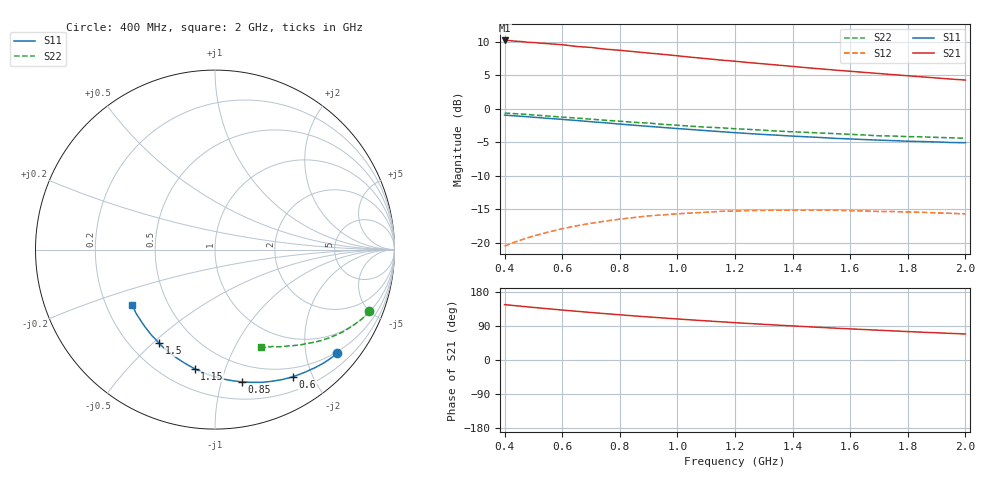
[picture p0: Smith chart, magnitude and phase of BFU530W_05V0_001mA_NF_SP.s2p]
! Filename:  P:\Prog\Test\Noise\ATS_data\Testdata_Net\06 Compressed Noise after Statistics\BFU530W_APM2013_09_A05_05p0V_001mA_NF_CM01_D.sf
! Date/Time: Tue 26/Mar/2013 18:06:06
! BFU530W_APM2013_09_A05_05p0V_1to25mA_NF_CM01_Bias1_R.sf
! Noise Parameter Data File
! BFU530W_APM2013_09_A05_05p0V_1to25mA_NF_CM01
! Date/time: Thu Mar 21 20:31:54 2013
! freq range =  0.4000 to  2.0000 GHz, 37 points
! bias range =  0.9950 to 25.0000 mA, 9 points
! bias supplies used: 1 1 0 0 0 0
! VAR bias_mode= 1  ! Specify V_out, I_out
! VAR bias_var = 1  ! Bias variable = I_out
! VAR V_out= 5.000000
! VAR I_out= 0.995000
! VAR V_in= 0.782600
! VAR I_in= 0.010101
! Device data file deembeded for feedlines and parallel
! Original file: \06 Compressed Noise after Statistics\BFU530W_APM2013_09_A05_05p0V_001mA_NF_CM01_R.sf
! Feed-files: PR019V01_070313_Feed1.s2p, PR019V01_070313_Feed2.s2p
! Parallel-file: PR019V01_070313_Par.s2p
# MHz S MA R 50
!  Freq-MHz  S11-mag  S11-arg  S21-mag  S21-arg  S12-mag  S12-arg  S22-mag  S22-arg
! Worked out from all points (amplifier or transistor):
!   37 points, 400 MHz to 2 GHz, reference 50 ohm
!   highest |S21| = 10.2 dB at 400 MHz (marker M1)
!   |S21| within 3 dB of that: start of sweep to 1.172 GHz
!   unconditionally stable (mu >= 1): nowhere
!   at 500 MHz: K = 0.20, MSG = 14.4 dB, |S12| = -19.0 dB
!   at 1.1 GHz: K = 0.41, MSG = 11.5 dB, |S12| = -15.5 dB
!   at 2 GHz: K = 0.77, MSG = 10.0 dB, |S12| = -15.7 dB
!   lowest NFmin = 0.48 dB at 420 MHz
!   S11 on the Smith chart (normalised r, x): 400 MHz: 0.46, -2.66; 600 MHz: 0.38, -1.72; 850 MHz: 0.34, -1.16; 1.15 GHz: 0.33, -0.79; 1.5 GHz: 0.32, -0.52; 2 GHz: 0.31, -0.28
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400  0.8945 -40.3  3.224 146.2  0.09419 64.3  0.9268 -21.8
420  0.8877 -42.2  3.212 144.6  0.09802 63.2  0.9211 -22.7
460  0.876 -46.0  3.163 141.7  0.1053 61.0  0.9099 -24.6
480  0.8694 -47.7  3.124 140.2  0.1087 59.9  0.9036 -25.5
500  0.8625 -49.6  3.111 138.7  0.112 58.9  0.8964 -26.3
600  0.8311 -58.5  2.998 131.8  0.127 54.0  0.8642 -30.5
650  0.8154 -62.6  2.908 128.6  0.1337 51.8  0.8504 -32.3
700  0.7982 -66.9  2.858 125.3  0.1395 49.5  0.834 -34.3
750  0.7834 -70.8  2.776 122.3  0.1449 47.6  0.8189 -35.9
800  0.7668 -74.7  2.723 119.3  0.1498 45.7  0.805 -37.6
850  0.7514 -78.7  2.659 116.4  0.1541 43.8  0.7903 -39.2
950  0.7236 -86.0  2.541 110.9  0.1611 40.4  0.7636 -42.2
1050  0.6977 -93.0  2.415 105.7  0.1665 37.4  0.7388 -44.9
1150  0.6732 -99.7  2.303 100.9  0.1713 34.7  0.7197 -47.2
1200  0.6618 -102.9  2.256 98.5  0.1721 33.5  0.7078 -48.7
1250  0.6512 -106.0  2.202 96.3  0.1739 32.3  0.6995 -49.6
1350  0.633 -112.1  2.11 92.0  0.1745 30.4  0.6796 -52.1
1500  0.6082 -120.8  1.977 85.9  0.1749 27.7  0.6574 -55.3
1600  0.5941 -126.4  1.899 82.1  0.1733 26.4  0.6429 -57.4
1750  0.577 -134.1  1.792 76.8  0.1707 25.2  0.6242 -60.2
1850  0.568 -139.1  1.724 73.4  0.1685 24.5  0.6158 -62.1
2000  0.557 -146.4  1.633 68.6  0.1638 24.5  0.6015 -65.0
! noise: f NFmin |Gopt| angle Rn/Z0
400  0.5358  0.6261  24.36  0.3103
460  0.5234  0.6349  27.94  0.3332
600  0.5889  0.6383  37.14  0.3289
800  0.543  0.6261  49.28  0.2894
1000  0.6921  0.6502  61.41  0.3076
1200  0.7441  0.6335  74.71  0.255
1400  0.788  0.6208  89.12  0.2023
1600  0.7562  0.5474  99.32  0.1568
1800  0.8933  0.5797  114.5  0.1448
2000  0.9541  0.5751  122.8  0.137
